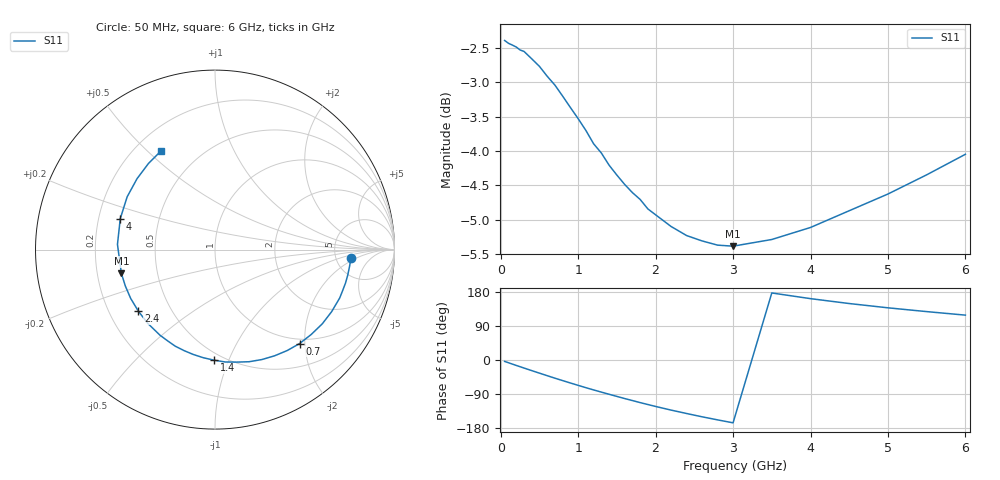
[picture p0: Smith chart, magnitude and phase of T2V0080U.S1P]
! SIEMENS Discrete & RF Semiconductors
! BAS70-04W
! Si Schottky Diode in SOT323
! IF = 0.08 mA
! S-Parameters:  November  1997
# GHz  S  MA  R  50
!  f  S11
! GHz  MAG  ANG
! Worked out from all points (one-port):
!   34 points, 50 MHz to 6 GHz, reference 50 ohm
!   lowest |S11| = -5.4 dB at 3 GHz (marker M1), VSWR 3.33, Z = 15.2 - j5.66 ohm
!   |S11| at or under -10 dB: nowhere
!   S11 on the Smith chart (normalised r, x): 50 MHz: 6.92, -1.60; 700 MHz: 0.91, -1.89; 1.4 GHz: 0.45, -0.89; 2.4 GHz: 0.32, -0.32; 4 GHz: 0.29, +0.15; 6 GHz: 0.30, +0.55
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0.05  0.759 -3.7
0.2  0.7507 -14.3
0.3  0.7452 -21.2
0.4  0.7361 -28.0
0.5  0.7268 -34.7
0.6  0.7149 -41.4
0.7  0.7044 -48.0
0.8  0.6915 -54.4
0.9  0.6785 -60.7
1  0.666 -66.9
1.1  0.6529 -73.1
1.3  0.6288 -84.8
1.4  0.6161 -90.5
1.5  0.606 -96.1
1.6  0.5967 -101.7
1.8  0.5819 -112.4
2  0.5671 -122.6
2.2  0.5562 -132.2
2.4  0.5478 -141.2
2.6  0.5429 -149.9
2.8  0.5391 -158.0
3  0.5382 -165.8
3.5  0.5442 176.9
4  0.5553 161.9
4.5  0.571 149.0
5  0.5872 137.7
5.5  0.6063 127.7
6  0.6275 118.4
